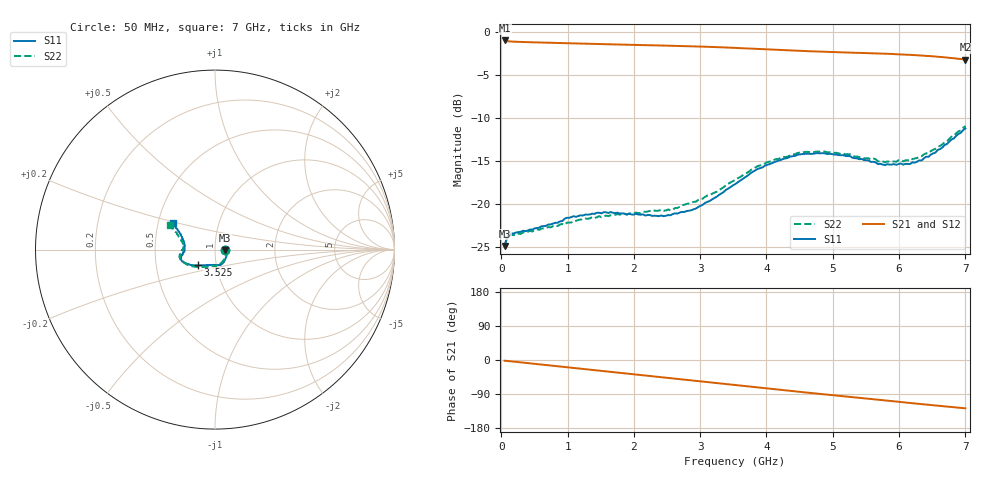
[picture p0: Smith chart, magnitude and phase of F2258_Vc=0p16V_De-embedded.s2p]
! Integrated Device Technology
! Corporate Headquarters
! 6024 Silver Creek Valley Road
! San Jose, CA 95138  USA
! Phone:  1-408-284-8200
! Toll Free:  1-800-223-1366
! Webpage:  http://www.idt.com/
! Timing and RF Division
! 515 Groton Road, Suite 102
! Westford, MA 01886-6024
! Device:  F2258
! Description: Voltage Variable RF Attenuator
! Frequency:  50.0 -  6000.00 MHz
! Package:  3x3 mm Thin QFN Plastic Package: 16 pin
! Ports:  2 RF, 2 DC
!  Pin  1  = NC
!  Pin  2  = NC
!  Pin  3  = RF2  = Port 2
!  Pin  4  = GND
!  Pin  5  = Vdd
!  Pin  6  = NC
!  Pin  7  = VCTRL
!  Pin  8  = NC
!  Pin  9  = GND
!  Pin 10  = RF1  = Port 1
!  Pin 11  = NC
!  Pin 12  = NC
!  Pin 13  = NC
!  Pin 14  = NC
!  Pin 15  = NC
!  Pin 16  = NC
! Vcntrl:  0.160 Volts
! Vdd:  +3.300 Volts
! Current:  1.076 mA
! Data:  The device was measured on a the F2258 evaluation board which has
!  individual transmission lines to the RF pins.  Data was collected
!  using a calibrated network analyzer.  The evaluation board was
!  de-embedded using a TRL calibration technique.
!  The reference plane is the edge of the package pin.
! Misc:  SN 10
!  Action Tracker AT0285
! Date Measured:  2014-12-10
! Date:  2016-01-13  MJV
! Note:
!  Integrated Device Technology supplies this data as a sample of measured
!  data at the package pin for this product.  Your particular data for this
!  product may vary.
!  Data was taken at 25 degrees C.
!  Integrated Device Technology reserves the right to change this data at anytime.
!Freq_(GHz)  S11M_(dB)  S11P_(deg)  S21M_(dB)  S21P_(deg)  S12M_(dB)  S12P_(deg)  S22M_(dB)  S22P_(deg)
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# GHz S dB R 50
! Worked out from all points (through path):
!   201 points, 50 MHz to 7 GHz, reference 50 ohm
!   highest |S21| = -0.96 dB at 50 MHz (marker M1); lowest = -3.2 dB at 7 GHz (marker M2)
!   group delay of S21, straight-line fit = 50.5 ps
!   lowest |S11| = -24.9 dB at 50 MHz (marker M3), VSWR 1.12, Z = 56 - j0.391 ohm
!   |S11| at or under -10 dB: start of sweep to end of sweep
!   |S22| runs from -24.9 to -10.9 dB; largest |S21 - S12| = 0.00036
!   S11 on the Smith chart (normalised r, x): 50 MHz: 1.12, -0.01; 3.525 GHz: 0.81, -0.14; 7 GHz: 0.60, +0.19
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0.05  -24.87 -3.5  -0.96 -1.9  -0.96 -1.9  -24.91 -3.1
0.08475  -23.90 -6.0  -1.03 -2.4  -1.03 -2.4  -23.97 -5.5
0.15425  -23.41 -9.3  -1.08 -3.6  -1.08 -3.6  -23.59 -9.4
0.71025  -22.38 -37.2  -1.22 -14.1  -1.22 -14.1  -22.69 -38.6
0.91875  -21.99 -46.9  -1.26 -18.0  -1.26 -18.0  -22.33 -50.4
0.98825  -21.60 -51.0  -1.27 -19.3  -1.27 -19.3  -22.17 -54.7
1.2315  -21.34 -59.3  -1.32 -23.8  -1.32 -23.8  -21.80 -63.7
1.6485  -20.94 -71.0  -1.41 -31.4  -1.41 -31.4  -21.31 -76.7
2.37825  -21.41 -92.4  -1.54 -44.8  -1.54 -44.8  -20.77 -94.3
2.552  -21.31 -98.4  -1.57 -48.0  -1.57 -48.0  -20.74 -99.6
2.93425  -20.53 -115.1  -1.65 -55.1  -1.65 -55.1  -19.73 -112.9
3.525  -17.70 -137.8  -1.82 -66.2  -1.82 -66.2  -17.21 -135.6
4.0115  -15.43 -151.4  -2.00 -75.2  -2.00 -75.2  -15.12 -151.0
4.46325  -14.28 -159.8  -2.16 -83.4  -2.16 -83.4  -14.07 -162.1
4.7065  -14.14 -163.0  -2.23 -87.7  -2.23 -87.7  -13.96 -166.3
5.2625  -14.43 -170.0  -2.38 -97.4  -2.38 -97.4  -14.21 -174.3
5.6795  -15.35 -176.8  -2.47 -104.6  -2.47 -104.6  -15.03 -179.7
5.85325  -15.41 179.0  -2.52 -107.8  -2.52 -107.8  -15.06 175.7
6.166  -15.34 171.2  -2.63 -113.4  -2.63 -113.4  -14.97 169.8
6.33975  -14.93 164.9  -2.71 -116.5  -2.71 -116.5  -14.43 165.4
6.722  -13.01 153.3  -2.94 -123.1  -2.95 -123.1  -12.71 156.4
7  -11.20 147.9  -3.19 -127.4  -3.19 -127.4  -10.92 151.5
